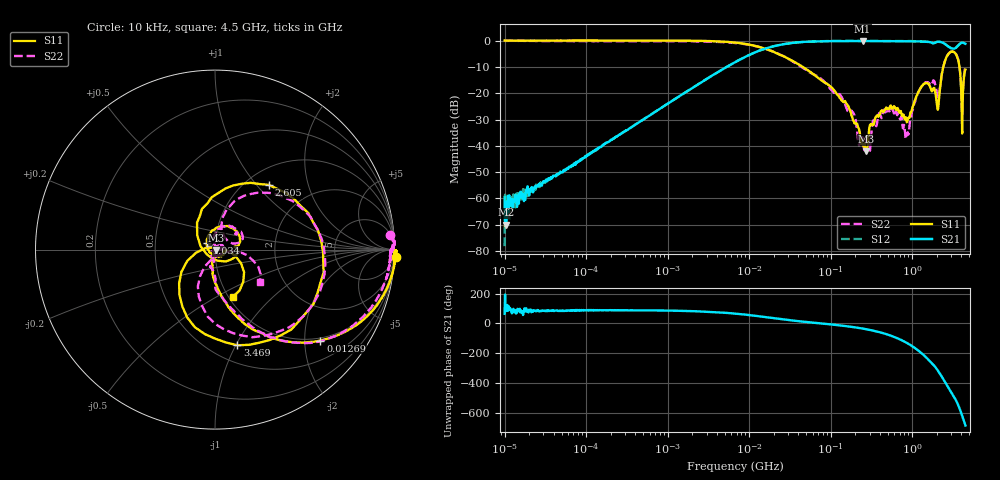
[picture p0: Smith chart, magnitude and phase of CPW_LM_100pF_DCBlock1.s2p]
!Siglent Technologies,SNA5004A,SNA5XCED5R0097,V1.0.0.2.10.R9
!Date: 2024-10-28 16:41:22
!Data & Calibration Information:
!Freq	S11:F2(ON)	S21:F2(ON)	S12:F2(ON)	S22:F2(ON)
# Hz S DB R 50
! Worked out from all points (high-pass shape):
!   1001 points, 10 kHz to 4.5 GHz, reference 50 ohm
!   highest |S21| = -0.12 dB at 246.9 MHz (marker M1); lowest = -70.0 dB at 10.4 kHz (marker M2)
!   |S21| within 3 dB of the highest: 15.37 MHz to end of sweep
!   lowest |S11| = -42.1 dB at 274 MHz (marker M3), VSWR 1.02, Z = 50.8 - j0.24 ohm
!   |S11| at or under -10 dB: 45.75 MHz to 2.409 GHz (2.364 GHz wide, 193 % of centre); 3.805 GHz to end of sweep
!   |S22| runs from -41.8 to 0.0 dB; largest |S21 - S12| = 0.018
!   S11 on the Smith chart (normalised r, x): 10 kHz: -10, -48; 12.69 MHz: 0.93, -2.37; 1.034 GHz: 0.91, +0.07; 2.605 GHz: 1.26, +1.16; 3.469 GHz: 0.67, -1.01; 4.5 GHz: 1.05, -0.60
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10000  0.07 -2.3  -59.63 64.1  -78.16 115.8  -0.17 4.9
10398.24  0.07 -2.0  -70.00 83.7  -63.00 79.7  -0.08 3.1
87919.76  0.07 -0.5  -45.22 90.4  -45.20 89.0  -0.18 -0.2
772988.4  0.04 -2.9  -26.24 86.7  -26.21 86.8  -0.21 -3.1
6708204  -0.69 -24.0  -8.18 65.9  -8.17 66.0  -0.85 -24.4
1.269444e7  -2.21 -40.8  -4.05 49.1  -4.05 49.3  -2.21 -41.3
5.897837e7  -12.37 -83.7  -0.33 5.7  -0.31 5.8  -12.52 -86.8
1.56561e8  -23.97 -105.7  -0.15 -18.7  -0.04 -18.5  -25.60 -101.1
2.469142e8  -39.59 -32.4  -0.12 -34.6  -0.09 -34.5  -36.68 -125.9
2.740134e8  -42.07 -17.5  -0.13 -39.2  -0.10 -39.0  -37.48 29.0
5.185364e8  -26.04 -11.0  -0.18 -78.1  -0.14 -77.8  -26.11 26.1
8.614985e8  -31.02 -128.5  -0.21 -131.3  -0.15 -131.0  -35.45 40.3
1.033712e9  -24.57 140.0  -0.23 -158.2  -0.19 -157.8  -25.44 96.1
1.358679e9  -16.71 64.0  -0.35 151.1  -0.32 151.6  -16.62 65.4
1.762711e9  -19.19 8.9  -0.88 88.1  -0.85 88.5  -16.15 39.6
2.228122e9  -16.22 130.3  -0.51 15.7  -0.49 16.2  -16.44 75.6
2.604819e9  -6.59 50.3  -1.54 -45.6  -1.54 -44.9  -6.61 40.5
3.00582e9  -4.17 -12.0  -2.86 -101.3  -2.84 -100.5  -4.14 -7.8
3.468552e9  -5.23 -76.9  -2.62 -159.9  -2.60 -159.0  -5.20 -61.2
3.750313e9  -8.74 -119.9  -1.50 158.5  -1.49 159.4  -8.51 -96.2
4.054962e9  -25.89 168.5  -0.76 107.9  -0.78 107.2  -24.90 -109.0
4.5e9  -11.01 -69.4  -1.17 33.5  -1.26 32.7  -10.24 -35.8
